(* Logix 5000 AddOnInstructionDefinition export HI6200_Faceplate_AOI; software revision 30.00; part 2 of 2 *)
(* tags used below, declared in another part *)
   Input_hi6200 : _0102:Hardy6200Series_F6857DC7:I:0;
   Output_hi6200 : _0102:Hardy6200Series_52E4DDE0:O:0;
   pm_4101 : REAL;   // Ref Weight
   pm_4182 : REAL;   // Span Weight
   pm_2082 : DINT;   // Averages
   pm_6302 : REAL;   // Auto Zero tolerance
   pm_2886 : REAL;   // Zero Tolerance
   pm_2887 : REAL;   // Motion tolerance
   pm_6183 : REAL;   // Tare Weight
   rd_filter_settings : BOOL;   // Read filter settings
   input_cmd_status : INT;   // Filtered Cmd Status
   rd_zero_tare_settings : BOOL;   // read zero and tare settings
   rd_setup1_settings : BOOL;   // read setup 1 settings
   rd_tradcal_settings : BOOL;   // program control bit to read hard cal ref weight
   write_tradcal_settings : BOOL;   // trigger write hard cal settings
   write_filter_settings : BOOL;   // trigger write filter settings
   write_zero_tare_settings : BOOL;   // trigger write zero and tare settings
   write_units_setting : BOOL;   // trigger write units of measure
   pm_2888 : REAL;   // Capacity
   rd_setup2_settings : BOOL;   // read setup 2 settings
   write_setup2_settings : BOOL;   // trigger write ins settup 2 settings
   write_setup1_settings : BOOL;   // trigger write ins setup 1 settings
   pm_2081w : DINT;   // write value setting for WAVERSAVER
   pm_6301w : DINT;   // write value setting for auto zero tracking enable
   pm_2881w : DINT;   // write value for setting units of measure
   pm_2882w : DINT;   // write value for setting decimal places
   pm_2883w : DINT;   // write value for setting grad size
   pm_4081w : DINT;   // write value for setting sensitivity value
   cmd_no : INT;   // cmd num holding register
   wr_hard_cal_ref_wt : BOOL;   // program control bit writing hard cal ref weight
   check_status_wr_traditional_ref : BOOL;   // operational code control bit write hard cal ref
   wr_span_wt : BOOL;   // program control bit writing span weight
   check_status_wr_span_wt : BOOL;   // operational code control bit write span weight
   ons_13 : BOOL;
   wr_waversaver : BOOL;   // program control bit writing WAVERSAVER
   check_status_wr_waversaver : BOOL;   // operational code control bit write WAVERSAVER
   wr_avgerages : BOOL;   // program control bit writing averages
   check_status_wr_averages : BOOL;   // operational code control bit write Averages
   wr_auto_zero_enable : BOOL;   // program control bit writing zuto zero enable
   check_status_wr_auto_zero_enable : BOOL;   // operational code control bit writing Auto Zero enable
   ons_14 : BOOL;
   wr_auto_zero_tolerance : BOOL;   // program control bit writing auto zero tolerance
   check_status_wr_auto_zero_tolerance : BOOL;   // operational code control bit writing Auto Zero tolerance
   wr_zero_tolerance : BOOL;   // program control bit writing zero tolerance
   check_status_wr_zero_tolerance : BOOL;   // operational code control bit write zero tolerance
   wr_units_measure : BOOL;   // program control bit writing units of measure
   ons_15 : BOOL;
   check_status_wr_units_measure : BOOL;   // operational code control bit write units of measure
   wr_motion_tolerance : BOOL;   // program control bit writing motion tolerance
   check_status_wr_motion_tolerance : BOOL;   // operational code control bit write motion tolerance
   wr_tare_weight : BOOL;   // program control bit writing tare weight
   check_status_wr_tare_weight : BOOL;   // operational code control bit write tare weight
   wr_sensitivity : BOOL;   // program control bit writing sensitivity
   check_status_wr_sensitivity : BOOL;   // operational code control bit write sensitivity
   wr_scale_capacity : BOOL;   // program control bit writing scale capacity
   check_status_wr_scale_capacity : BOOL;   // operational code control bit write scale capacity
   ons_17 : BOOL;
   wr_decimal_point : BOOL;   // program control bit writing decimal point
   check_status_wr_decimal_point : BOOL;   // operational code control bit writing decimal points
   wr_grad_size : BOOL;   // program control bit writing grad size
   check_status_wr_grads_size : BOOL;   // operational code control bit write grad size
   ons_18 : BOOL;
(* HI6200_Faceplate_AOI, continued *)

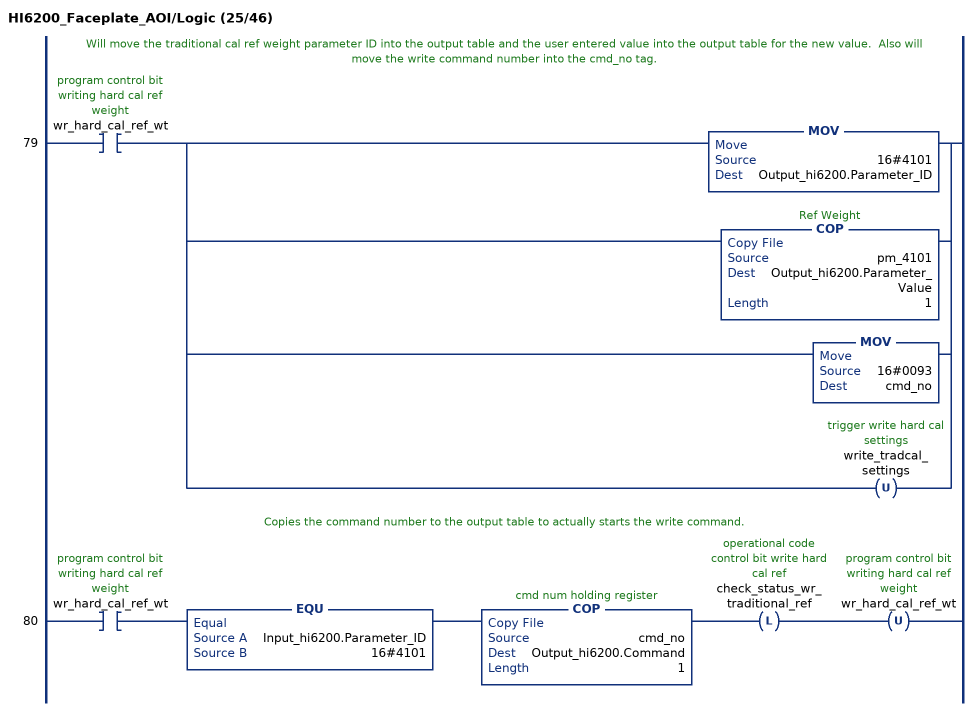
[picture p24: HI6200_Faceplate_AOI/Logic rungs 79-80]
   // Will move the traditional cal ref weight parameter ID into the output table and the user entered value into the output table for the new value.  Also will move the write command number into the cmd_no tag.
   79: XIC(wr_hard_cal_ref_wt)[MOV(16#4101,Output_hi6200.Parameter_ID) ,COP(pm_4101,Output_hi6200.Parameter_Value,1) ,MOV(16#0093,cmd_no) ,OTU(write_tradcal_settings) ];
   // Copies the command number to the output table to actually starts the write command.
   80: XIC(wr_hard_cal_ref_wt)EQU(Input_hi6200.Parameter_ID,16#4101)COP(cmd_no,Output_hi6200.Command,1)OTL(check_status_wr_traditional_ref)OTU(wr_hard_cal_ref_wt);
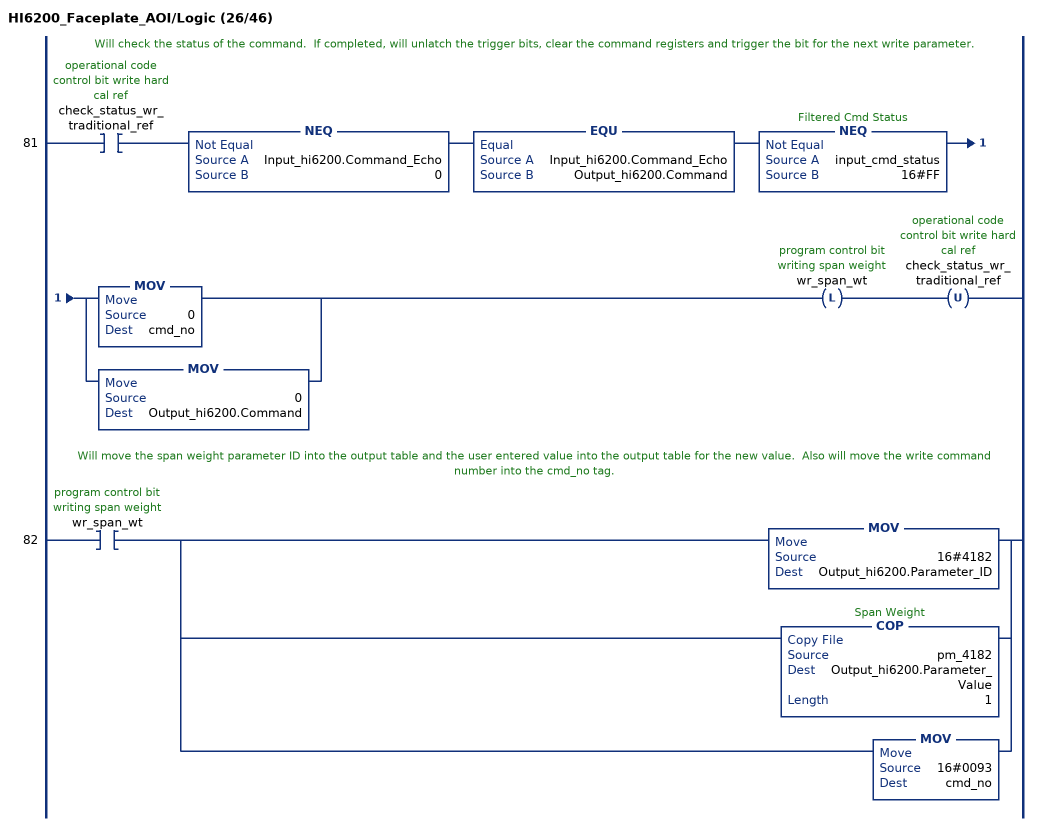
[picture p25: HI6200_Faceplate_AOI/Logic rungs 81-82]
   // Will check the status of the command.  If completed, will unlatch the trigger bits, clear the command registers and trigger the bit for the next write parameter.
   81: XIC(check_status_wr_traditional_ref)NEQ(Input_hi6200.Command_Echo,0)EQU(Input_hi6200.Command_Echo,Output_hi6200.Command)NEQ(input_cmd_status,16#FF)[MOV(0,cmd_no) ,MOV(0,Output_hi6200.Command) ]OTL(wr_span_wt)OTU(check_status_wr_traditional_ref);
   // Will move the span weight parameter ID into the output table and the user entered value into the output table for the new value.  Also will move the write command number into the cmd_no tag.
   82: XIC(wr_span_wt)[MOV(16#4182,Output_hi6200.Parameter_ID) ,COP(pm_4182,Output_hi6200.Parameter_Value,1) ,MOV(16#0093,cmd_no) ];
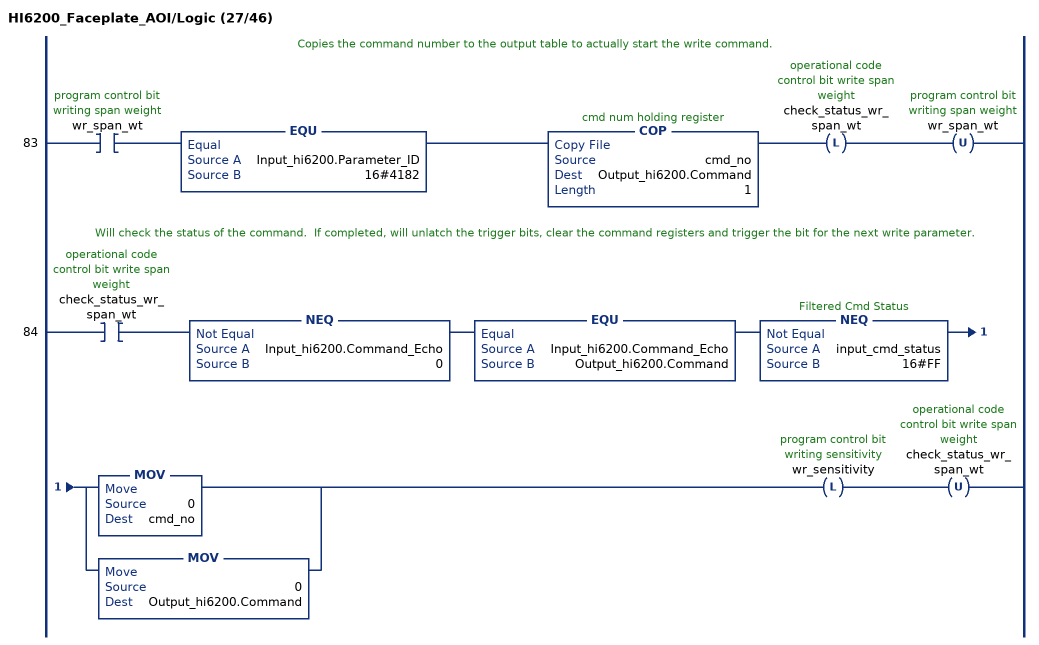
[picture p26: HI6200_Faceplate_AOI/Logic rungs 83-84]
   // Copies the command number to the output table to actually start the write command.
   83: XIC(wr_span_wt)EQU(Input_hi6200.Parameter_ID,16#4182)COP(cmd_no,Output_hi6200.Command,1)OTL(check_status_wr_span_wt)OTU(wr_span_wt);
   // Will check the status of the command.  If completed, will unlatch the trigger bits, clear the command registers and trigger the bit for the next write parameter.
   84: XIC(check_status_wr_span_wt)NEQ(Input_hi6200.Command_Echo,0)EQU(Input_hi6200.Command_Echo,Output_hi6200.Command)NEQ(input_cmd_status,16#FF)[MOV(0,cmd_no) ,MOV(0,Output_hi6200.Command) ]OTL(wr_sensitivity)OTU(check_status_wr_span_wt);
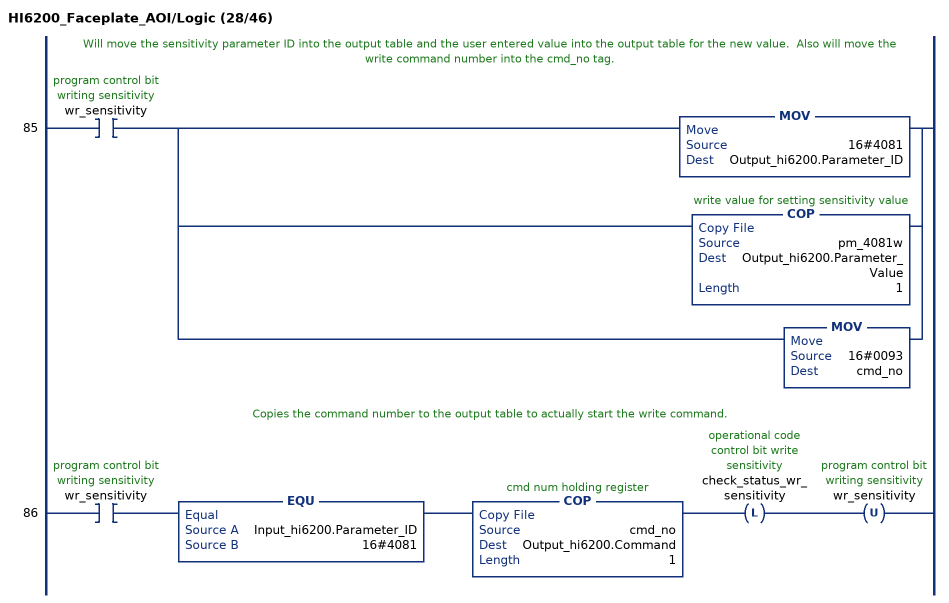
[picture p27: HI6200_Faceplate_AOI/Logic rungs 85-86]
   // Will move the sensitivity parameter ID into the output table and the user entered value into the output table for the new value.  Also will move the write command number into the cmd_no tag.
   85: XIC(wr_sensitivity)[MOV(16#4081,Output_hi6200.Parameter_ID) ,COP(pm_4081w,Output_hi6200.Parameter_Value,1) ,MOV(16#0093,cmd_no) ];
   // Copies the command number to the output table to actually start the write command.
   86: XIC(wr_sensitivity)EQU(Input_hi6200.Parameter_ID,16#4081)COP(cmd_no,Output_hi6200.Command,1)OTL(check_status_wr_sensitivity)OTU(wr_sensitivity);
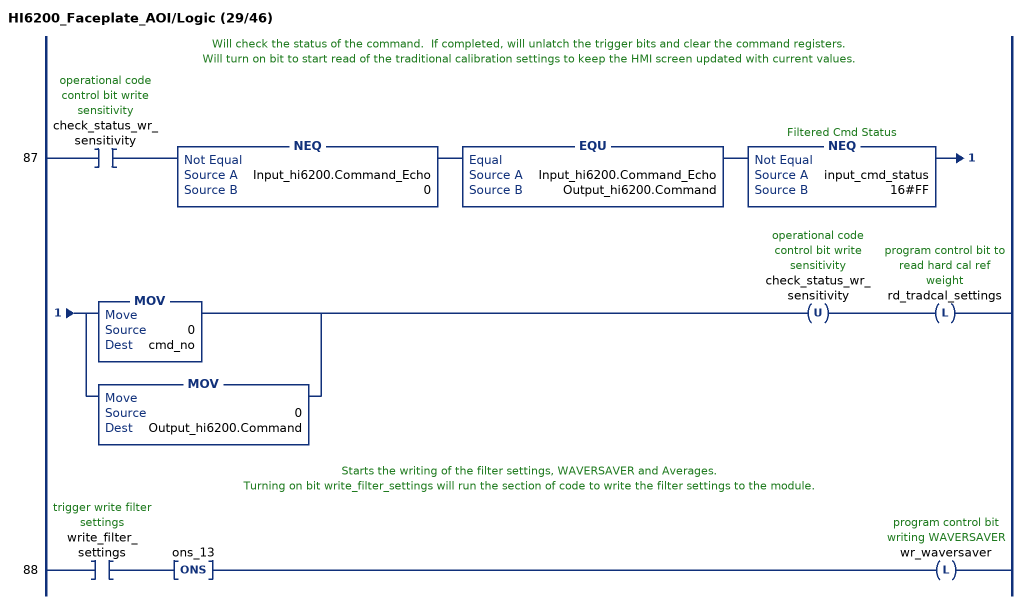
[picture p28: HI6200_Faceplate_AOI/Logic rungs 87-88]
   // Will check the status of the command.  If completed, will unlatch the trigger bits and clear the command registers.
   // Will turn on bit to start read of the traditional calibration settings to keep the HMI screen updated with current values.
   87: XIC(check_status_wr_sensitivity)NEQ(Input_hi6200.Command_Echo,0)EQU(Input_hi6200.Command_Echo,Output_hi6200.Command)NEQ(input_cmd_status,16#FF)[MOV(0,cmd_no) ,MOV(0,Output_hi6200.Command) ]OTU(check_status_wr_sensitivity)OTL(rd_tradcal_settings);
   // Starts the writing of the filter settings, WAVERSAVER and Averages.
   // Turning on bit write_filter_settings will run the section of code to write the filter settings to the module.
   88: XIC(write_filter_settings)ONS(ons_13)OTL(wr_waversaver);
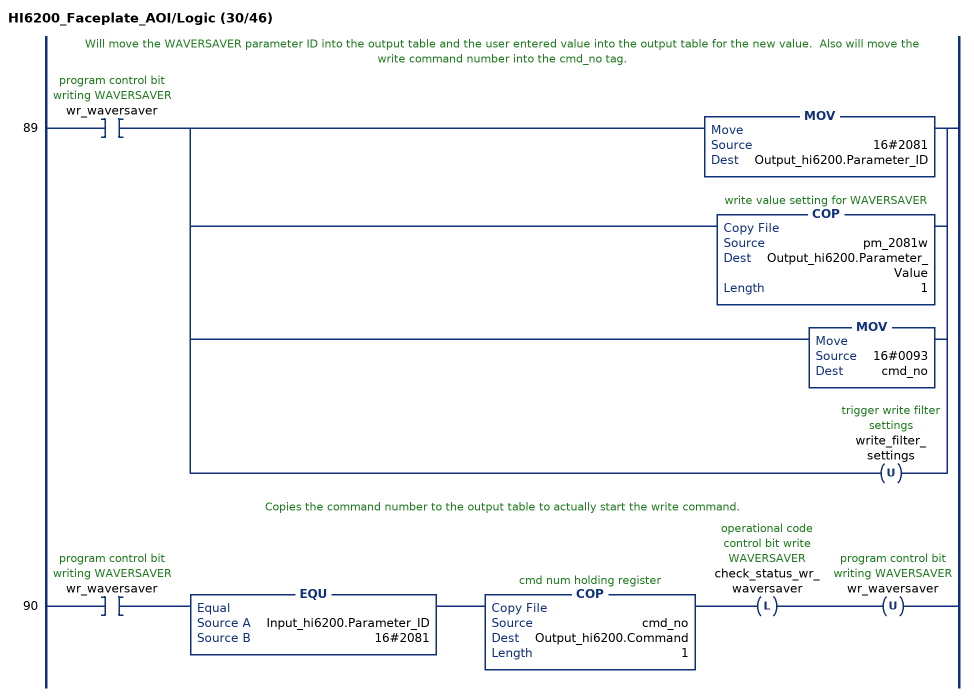
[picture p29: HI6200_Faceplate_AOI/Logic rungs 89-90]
   // Will move the WAVERSAVER parameter ID into the output table and the user entered value into the output table for the new value.  Also will move the write command number into the cmd_no tag.
   89: XIC(wr_waversaver)[MOV(16#2081,Output_hi6200.Parameter_ID) ,COP(pm_2081w,Output_hi6200.Parameter_Value,1) ,MOV(16#0093,cmd_no) ,OTU(write_filter_settings) ];
   // Copies the command number to the output table to actually start the write command.
   90: XIC(wr_waversaver)EQU(Input_hi6200.Parameter_ID,16#2081)COP(cmd_no,Output_hi6200.Command,1)OTL(check_status_wr_waversaver)OTU(wr_waversaver);
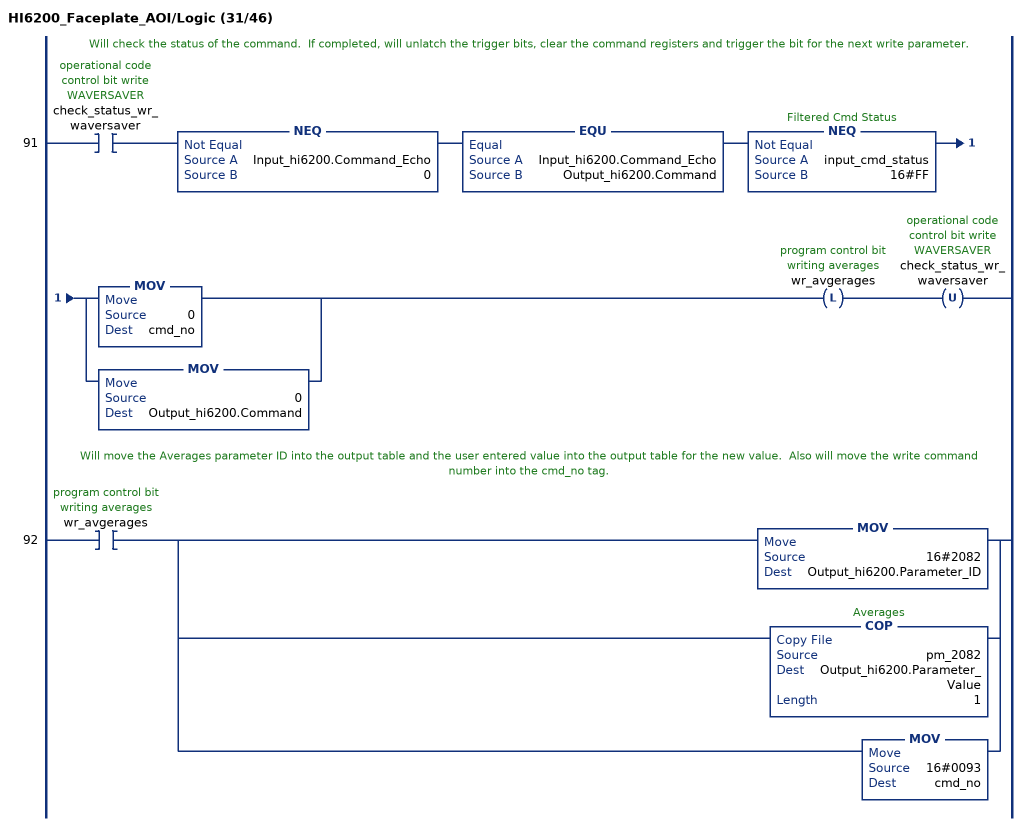
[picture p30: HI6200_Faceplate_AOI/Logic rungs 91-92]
   // Will check the status of the command.  If completed, will unlatch the trigger bits, clear the command registers and trigger the bit for the next write parameter.
   91: XIC(check_status_wr_waversaver)NEQ(Input_hi6200.Command_Echo,0)EQU(Input_hi6200.Command_Echo,Output_hi6200.Command)NEQ(input_cmd_status,16#FF)[MOV(0,cmd_no) ,MOV(0,Output_hi6200.Command) ]OTL(wr_avgerages)OTU(check_status_wr_waversaver);
   // Will move the Averages parameter ID into the output table and the user entered value into the output table for the new value.  Also will move the write command number into the cmd_no tag.
   92: XIC(wr_avgerages)[MOV(16#2082,Output_hi6200.Parameter_ID) ,COP(pm_2082,Output_hi6200.Parameter_Value,1) ,MOV(16#0093,cmd_no) ];
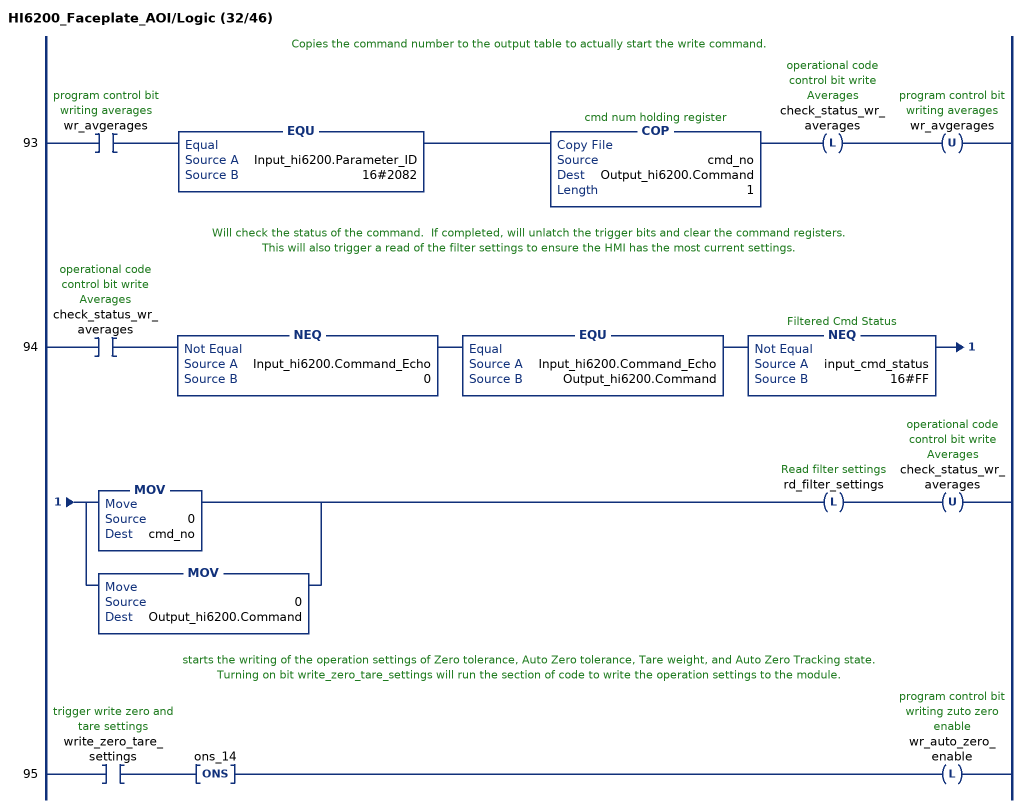
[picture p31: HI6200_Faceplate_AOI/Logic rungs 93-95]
   // Copies the command number to the output table to actually start the write command.
   93: XIC(wr_avgerages)EQU(Input_hi6200.Parameter_ID,16#2082)COP(cmd_no,Output_hi6200.Command,1)OTL(check_status_wr_averages)OTU(wr_avgerages);
   // Will check the status of the command.  If completed, will unlatch the trigger bits and clear the command registers.
   // This will also trigger a read of the filter settings to ensure the HMI has the most current settings.
   94: XIC(check_status_wr_averages)NEQ(Input_hi6200.Command_Echo,0)EQU(Input_hi6200.Command_Echo,Output_hi6200.Command)NEQ(input_cmd_status,16#FF)[MOV(0,cmd_no) ,MOV(0,Output_hi6200.Command) ]OTL(rd_filter_settings)OTU(check_status_wr_averages);
   // starts the writing of the operation settings of Zero tolerance, Auto Zero tolerance, Tare weight, and Auto Zero Tracking state.
   // Turning on bit write_zero_tare_settings will run the section of code to write the operation settings to the module.
   95: XIC(write_zero_tare_settings)ONS(ons_14)OTL(wr_auto_zero_enable);
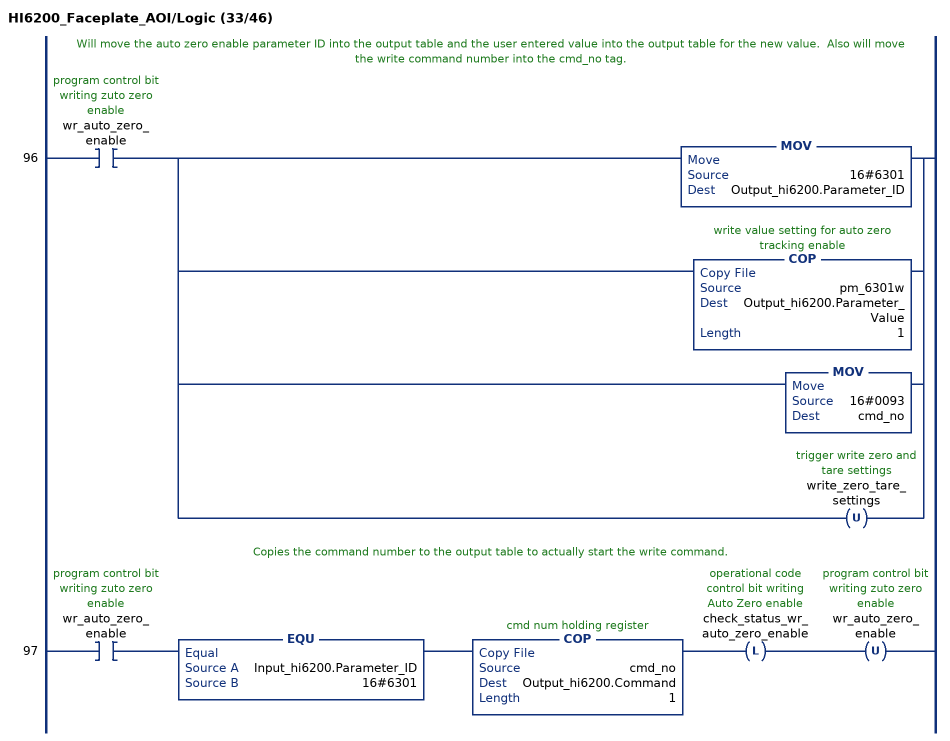
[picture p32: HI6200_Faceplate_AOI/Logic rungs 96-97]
   // Will move the auto zero enable parameter ID into the output table and the user entered value into the output table for the new value.  Also will move the write command number into the cmd_no tag.
   96: XIC(wr_auto_zero_enable)[MOV(16#6301,Output_hi6200.Parameter_ID) ,COP(pm_6301w,Output_hi6200.Parameter_Value,1) ,MOV(16#0093,cmd_no) ,OTU(write_zero_tare_settings) ];
   // Copies the command number to the output table to actually start the write command.
   97: XIC(wr_auto_zero_enable)EQU(Input_hi6200.Parameter_ID,16#6301)COP(cmd_no,Output_hi6200.Command,1)OTL(check_status_wr_auto_zero_enable)OTU(wr_auto_zero_enable);
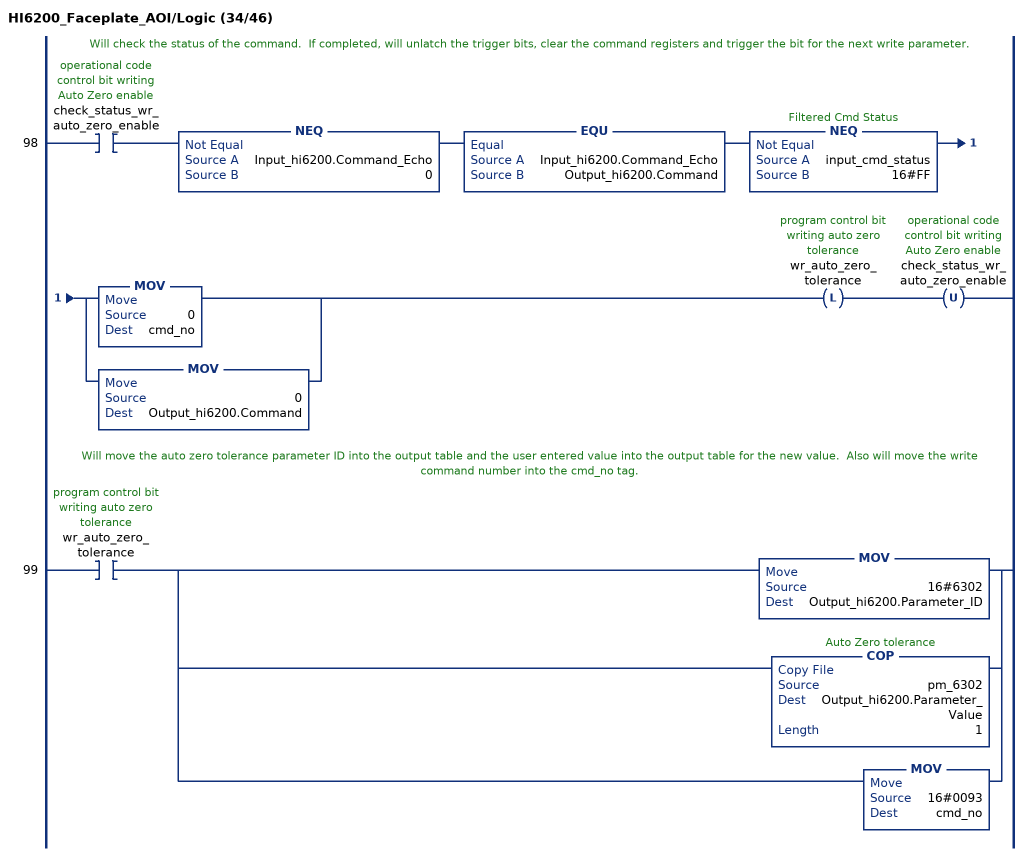
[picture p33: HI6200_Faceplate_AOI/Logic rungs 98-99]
   // Will check the status of the command.  If completed, will unlatch the trigger bits, clear the command registers and trigger the bit for the next write parameter.
   98: XIC(check_status_wr_auto_zero_enable)NEQ(Input_hi6200.Command_Echo,0)EQU(Input_hi6200.Command_Echo,Output_hi6200.Command)NEQ(input_cmd_status,16#FF)[MOV(0,cmd_no) ,MOV(0,Output_hi6200.Command) ]OTL(wr_auto_zero_tolerance)OTU(check_status_wr_auto_zero_enable);
   // Will move the auto zero tolerance parameter ID into the output table and the user entered value into the output table for the new value.  Also will move the write command number into the cmd_no tag.
   99: XIC(wr_auto_zero_tolerance)[MOV(16#6302,Output_hi6200.Parameter_ID) ,COP(pm_6302,Output_hi6200.Parameter_Value,1) ,MOV(16#0093,cmd_no) ];
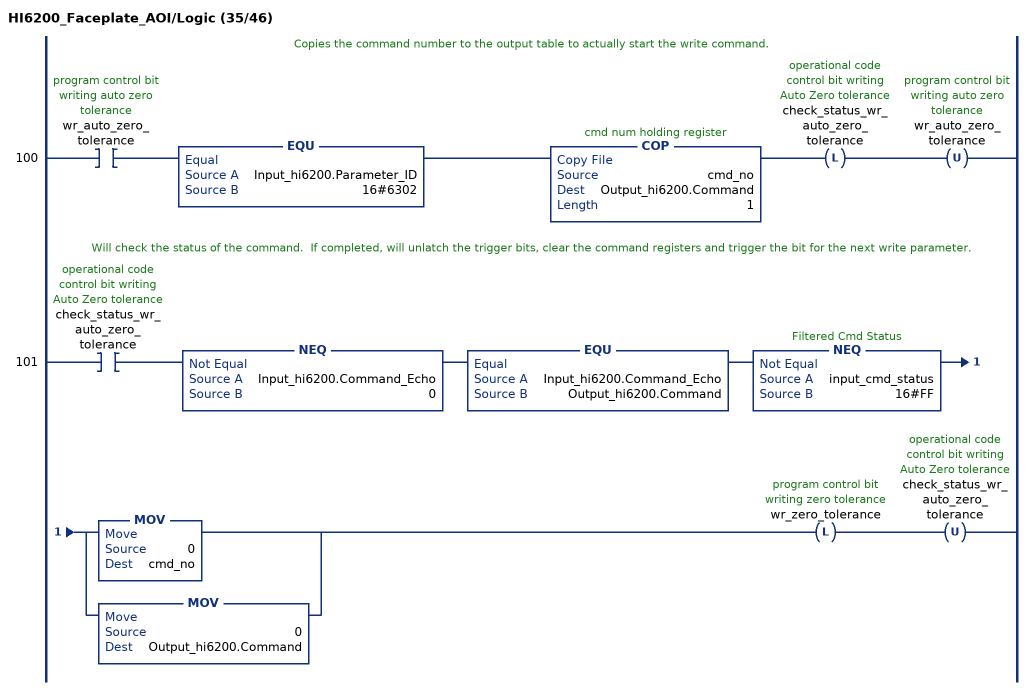
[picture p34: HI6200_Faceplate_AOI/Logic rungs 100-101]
   // Copies the command number to the output table to actually start the write command.
   100: XIC(wr_auto_zero_tolerance)EQU(Input_hi6200.Parameter_ID,16#6302)COP(cmd_no,Output_hi6200.Command,1)OTL(check_status_wr_auto_zero_tolerance)OTU(wr_auto_zero_tolerance);
   // Will check the status of the command.  If completed, will unlatch the trigger bits, clear the command registers and trigger the bit for the next write parameter.
   101: XIC(check_status_wr_auto_zero_tolerance)NEQ(Input_hi6200.Command_Echo,0)EQU(Input_hi6200.Command_Echo,Output_hi6200.Command)NEQ(input_cmd_status,16#FF)[MOV(0,cmd_no) ,MOV(0,Output_hi6200.Command) ]OTL(wr_zero_tolerance)OTU(check_status_wr_auto_zero_tolerance);
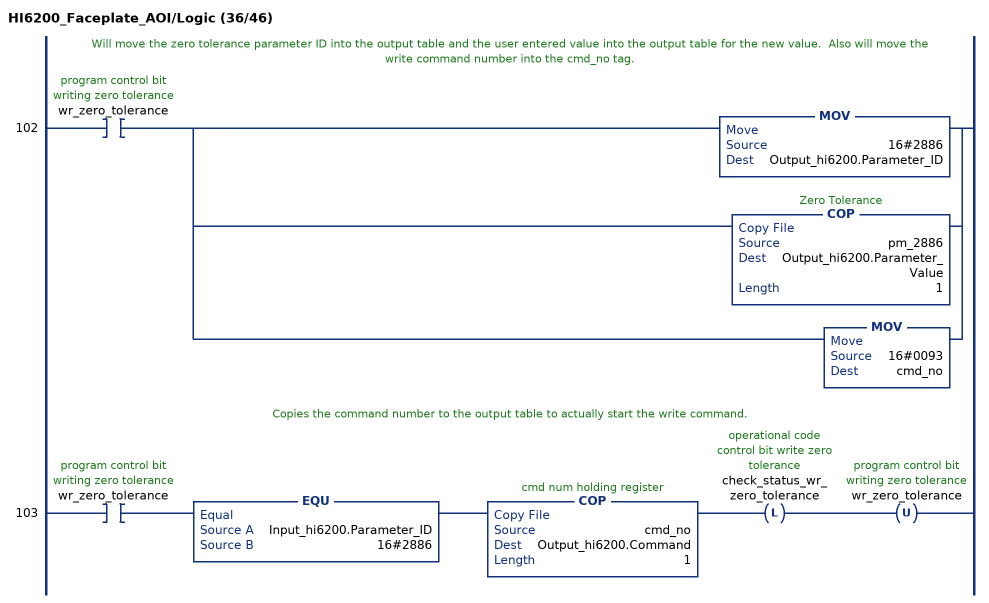
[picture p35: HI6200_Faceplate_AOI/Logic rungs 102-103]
   // Will move the zero tolerance parameter ID into the output table and the user entered value into the output table for the new value.  Also will move the write command number into the cmd_no tag.
   102: XIC(wr_zero_tolerance)[MOV(16#2886,Output_hi6200.Parameter_ID) ,COP(pm_2886,Output_hi6200.Parameter_Value,1) ,MOV(16#0093,cmd_no) ];
   // Copies the command number to the output table to actually start the write command.
   103: XIC(wr_zero_tolerance)EQU(Input_hi6200.Parameter_ID,16#2886)COP(cmd_no,Output_hi6200.Command,1)OTL(check_status_wr_zero_tolerance)OTU(wr_zero_tolerance);
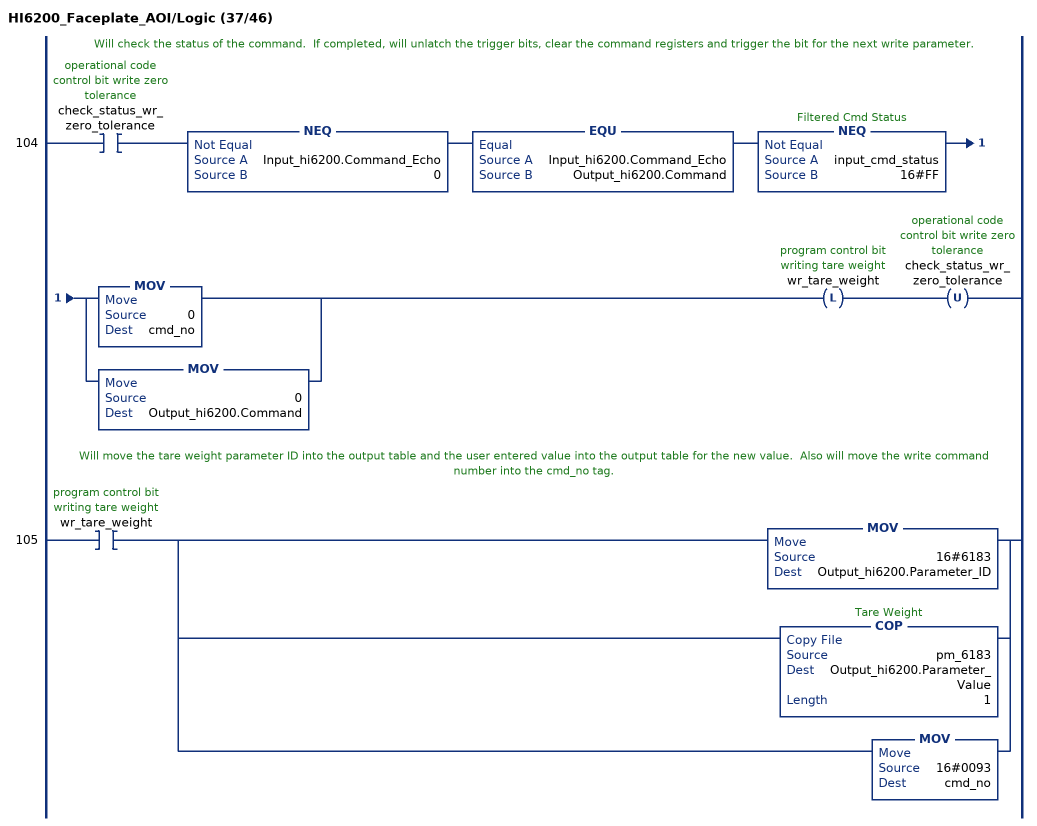
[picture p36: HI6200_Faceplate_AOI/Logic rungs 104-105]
   // Will check the status of the command.  If completed, will unlatch the trigger bits, clear the command registers and trigger the bit for the next write parameter.
   104: XIC(check_status_wr_zero_tolerance)NEQ(Input_hi6200.Command_Echo,0)EQU(Input_hi6200.Command_Echo,Output_hi6200.Command)NEQ(input_cmd_status,16#FF)[MOV(0,cmd_no) ,MOV(0,Output_hi6200.Command) ]OTL(wr_tare_weight)OTU(check_status_wr_zero_tolerance);
   // Will move the tare weight parameter ID into the output table and the user entered value into the output table for the new value.  Also will move the write command number into the cmd_no tag.
   105: XIC(wr_tare_weight)[MOV(16#6183,Output_hi6200.Parameter_ID) ,COP(pm_6183,Output_hi6200.Parameter_Value,1) ,MOV(16#0093,cmd_no) ];
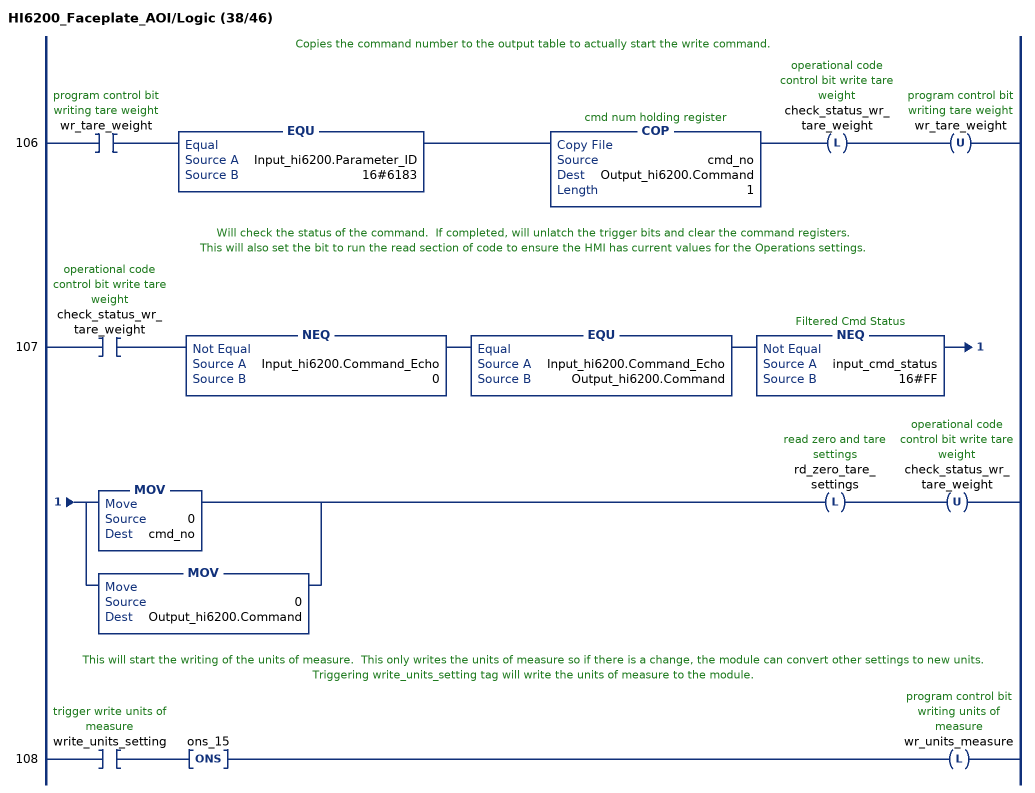
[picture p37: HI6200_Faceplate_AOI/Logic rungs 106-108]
   // Copies the command number to the output table to actually start the write command.
   106: XIC(wr_tare_weight)EQU(Input_hi6200.Parameter_ID,16#6183)COP(cmd_no,Output_hi6200.Command,1)OTL(check_status_wr_tare_weight)OTU(wr_tare_weight);
   // Will check the status of the command.  If completed, will unlatch the trigger bits and clear the command registers.
   // This will also set the bit to run the read section of code to ensure the HMI has current values for the Operations settings.
   107: XIC(check_status_wr_tare_weight)NEQ(Input_hi6200.Command_Echo,0)EQU(Input_hi6200.Command_Echo,Output_hi6200.Command)NEQ(input_cmd_status,16#FF)[MOV(0,cmd_no) ,MOV(0,Output_hi6200.Command) ]OTL(rd_zero_tare_settings)OTU(check_status_wr_tare_weight);
   // This will start the writing of the units of measure.  This only writes the units of measure so if there is a change, the module can convert other settings to new units.
   // Triggering write_units_setting tag will write the units of measure to the module.
   108: XIC(write_units_setting)ONS(ons_15)OTL(wr_units_measure);
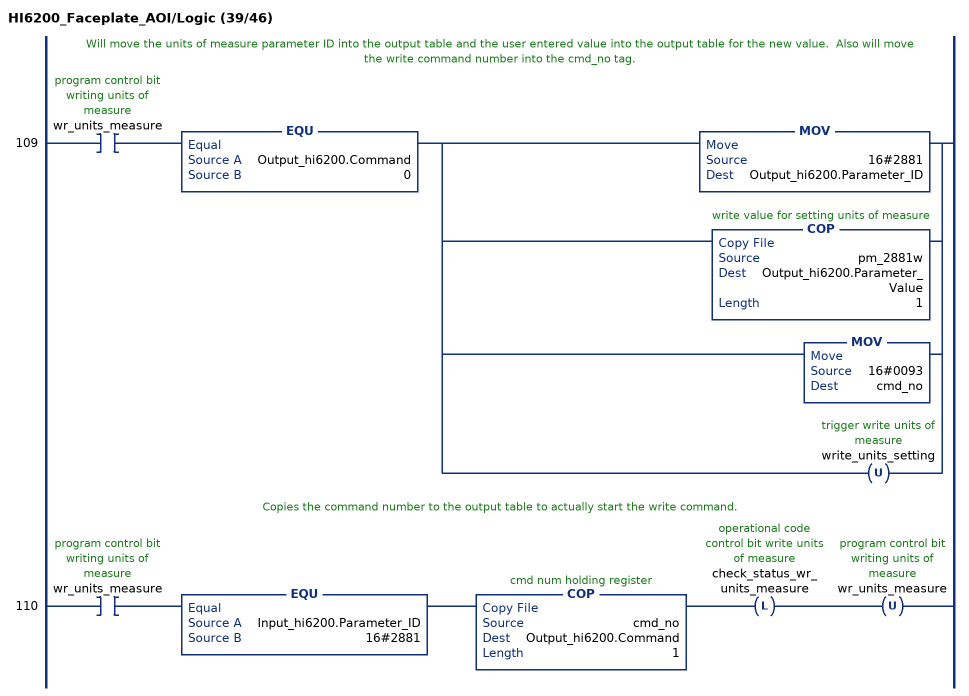
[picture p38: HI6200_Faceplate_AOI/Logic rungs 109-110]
   // Will move the units of measure parameter ID into the output table and the user entered value into the output table for the new value.  Also will move the write command number into the cmd_no tag.
   109: XIC(wr_units_measure)EQU(Output_hi6200.Command,0)[MOV(16#2881,Output_hi6200.Parameter_ID) ,COP(pm_2881w,Output_hi6200.Parameter_Value,1) ,MOV(16#0093,cmd_no) ,OTU(write_units_setting) ];
   // Copies the command number to the output table to actually start the write command.
   110: XIC(wr_units_measure)EQU(Input_hi6200.Parameter_ID,16#2881)COP(cmd_no,Output_hi6200.Command,1)OTL(check_status_wr_units_measure)OTU(wr_units_measure);
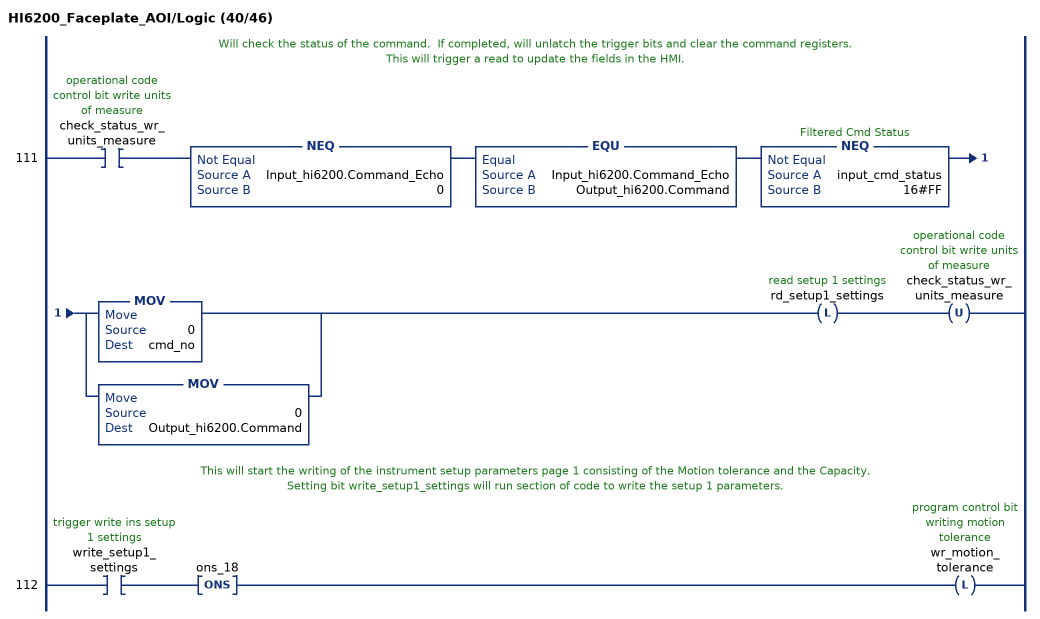
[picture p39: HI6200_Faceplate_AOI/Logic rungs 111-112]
   // Will check the status of the command.  If completed, will unlatch the trigger bits and clear the command registers.
   // This will trigger a read to update the fields in the HMI.
   111: XIC(check_status_wr_units_measure)NEQ(Input_hi6200.Command_Echo,0)EQU(Input_hi6200.Command_Echo,Output_hi6200.Command)NEQ(input_cmd_status,16#FF)[MOV(0,cmd_no) ,MOV(0,Output_hi6200.Command) ]OTL(rd_setup1_settings)OTU(check_status_wr_units_measure);
   // This will start the writing of the instrument setup parameters page 1 consisting of the Motion tolerance and the Capacity.
   // Setting bit write_setup1_settings will run section of code to write the setup 1 parameters.
   112: XIC(write_setup1_settings)ONS(ons_18)OTL(wr_motion_tolerance);
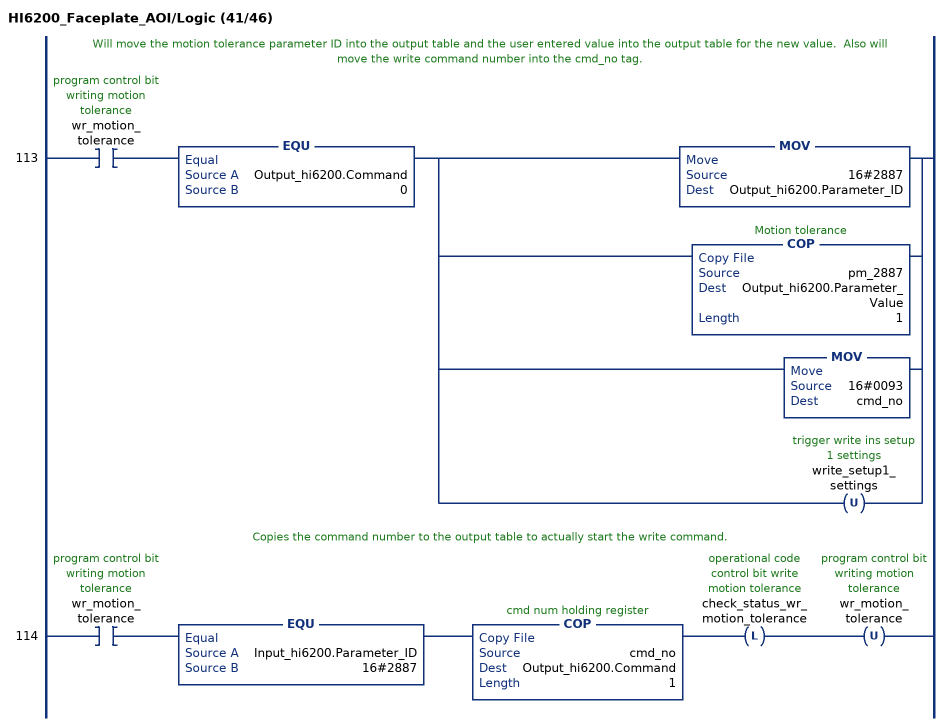
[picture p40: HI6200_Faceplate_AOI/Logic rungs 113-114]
   // Will move the motion tolerance parameter ID into the output table and the user entered value into the output table for the new value.  Also will move the write command number into the cmd_no tag.
   113: XIC(wr_motion_tolerance)EQU(Output_hi6200.Command,0)[MOV(16#2887,Output_hi6200.Parameter_ID) ,COP(pm_2887,Output_hi6200.Parameter_Value,1) ,MOV(16#0093,cmd_no) ,OTU(write_setup1_settings) ];
   // Copies the command number to the output table to actually start the write command.
   114: XIC(wr_motion_tolerance)EQU(Input_hi6200.Parameter_ID,16#2887)COP(cmd_no,Output_hi6200.Command,1)OTL(check_status_wr_motion_tolerance)OTU(wr_motion_tolerance);
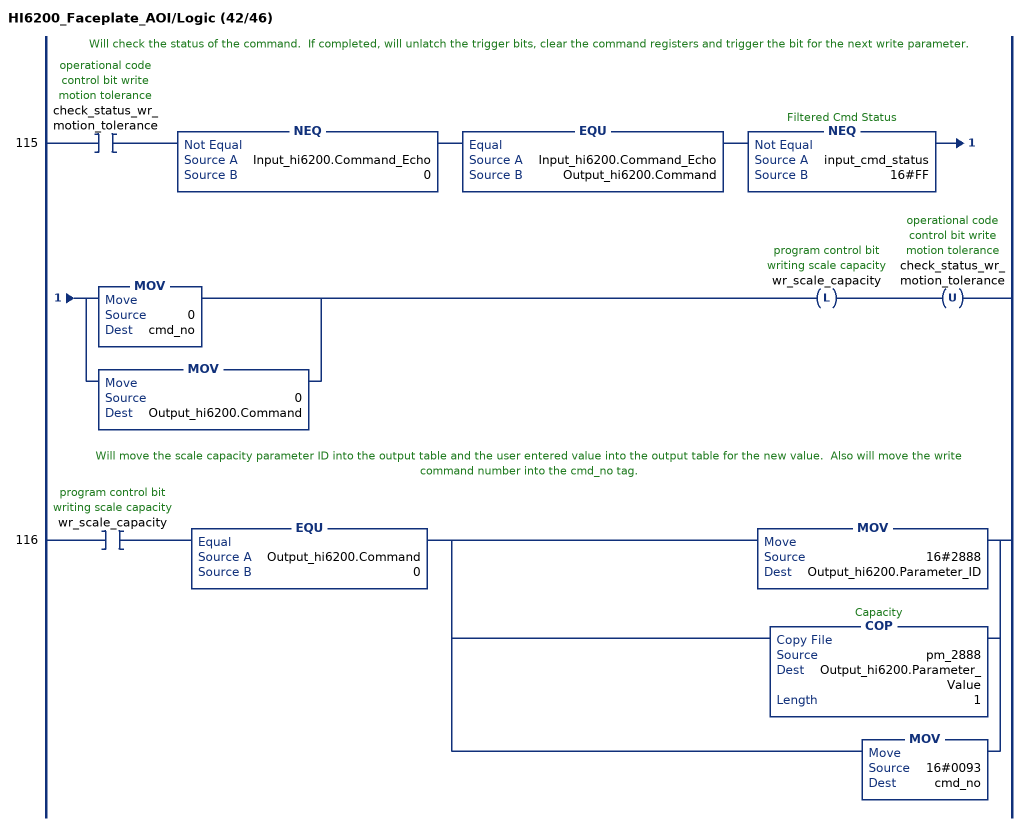
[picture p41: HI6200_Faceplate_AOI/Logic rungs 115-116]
   // Will check the status of the command.  If completed, will unlatch the trigger bits, clear the command registers and trigger the bit for the next write parameter.
   115: XIC(check_status_wr_motion_tolerance)NEQ(Input_hi6200.Command_Echo,0)EQU(Input_hi6200.Command_Echo,Output_hi6200.Command)NEQ(input_cmd_status,16#FF)[MOV(0,cmd_no) ,MOV(0,Output_hi6200.Command) ]OTL(wr_scale_capacity)OTU(check_status_wr_motion_tolerance);
   // Will move the scale capacity parameter ID into the output table and the user entered value into the output table for the new value.  Also will move the write command number into the cmd_no tag.
   116: XIC(wr_scale_capacity)EQU(Output_hi6200.Command,0)[MOV(16#2888,Output_hi6200.Parameter_ID) ,COP(pm_2888,Output_hi6200.Parameter_Value,1) ,MOV(16#0093,cmd_no) ];
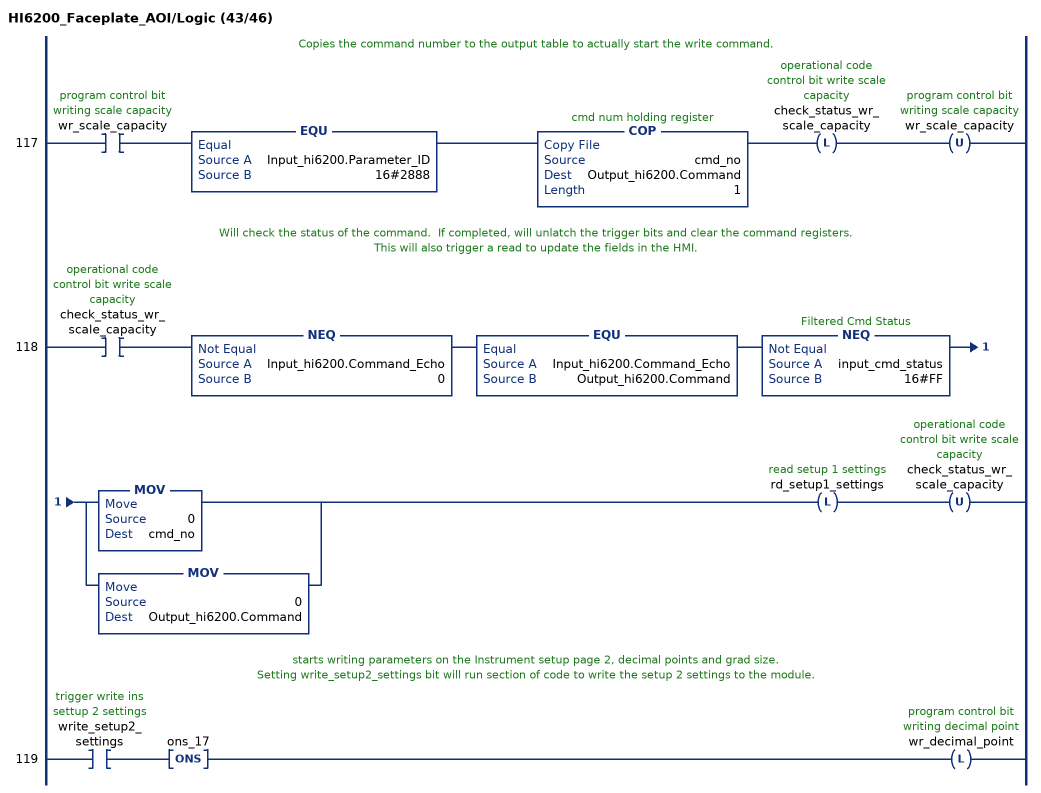
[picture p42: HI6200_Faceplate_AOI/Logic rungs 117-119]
   // Copies the command number to the output table to actually start the write command.
   117: XIC(wr_scale_capacity)EQU(Input_hi6200.Parameter_ID,16#2888)COP(cmd_no,Output_hi6200.Command,1)OTL(check_status_wr_scale_capacity)OTU(wr_scale_capacity);
   // Will check the status of the command.  If completed, will unlatch the trigger bits and clear the command registers.
   // This will also trigger a read to update the fields in the HMI.
   118: XIC(check_status_wr_scale_capacity)NEQ(Input_hi6200.Command_Echo,0)EQU(Input_hi6200.Command_Echo,Output_hi6200.Command)NEQ(input_cmd_status,16#FF)[MOV(0,cmd_no) ,MOV(0,Output_hi6200.Command) ]OTL(rd_setup1_settings)OTU(check_status_wr_scale_capacity);
   // starts writing parameters on the Instrument setup page 2, decimal points and grad size.
   // Setting write_setup2_settings bit will run section of code to write the setup 2 settings to the module.
   119: XIC(write_setup2_settings)ONS(ons_17)OTL(wr_decimal_point);
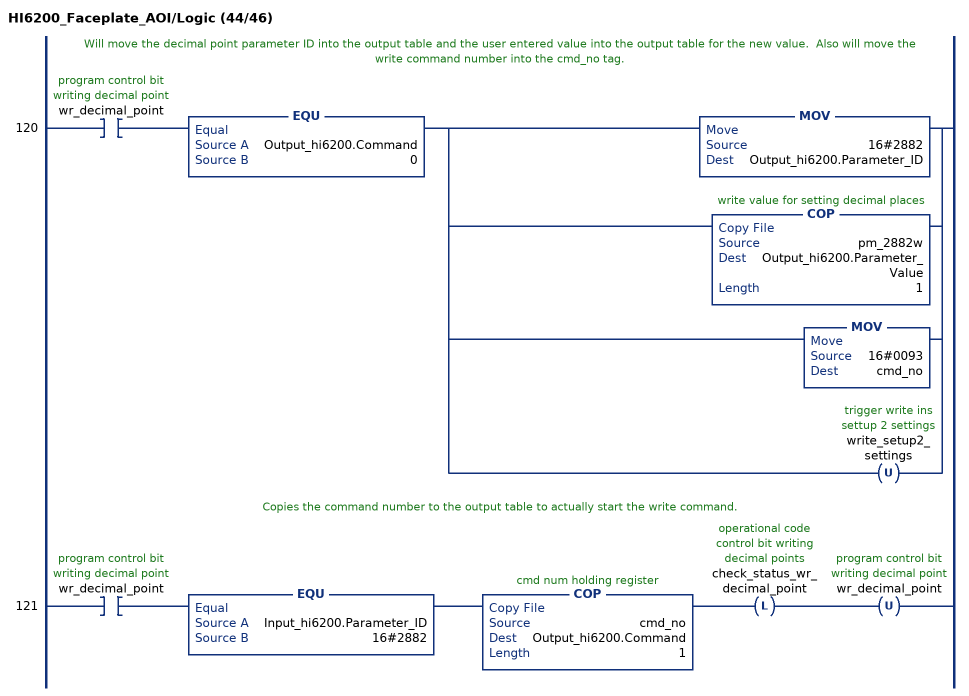
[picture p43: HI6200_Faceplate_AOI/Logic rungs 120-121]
   // Will move the decimal point parameter ID into the output table and the user entered value into the output table for the new value.  Also will move the write command number into the cmd_no tag.
   120: XIC(wr_decimal_point)EQU(Output_hi6200.Command,0)[MOV(16#2882,Output_hi6200.Parameter_ID) ,COP(pm_2882w,Output_hi6200.Parameter_Value,1) ,MOV(16#0093,cmd_no) ,OTU(write_setup2_settings) ];
   // Copies the command number to the output table to actually start the write command.
   121: XIC(wr_decimal_point)EQU(Input_hi6200.Parameter_ID,16#2882)COP(cmd_no,Output_hi6200.Command,1)OTL(check_status_wr_decimal_point)OTU(wr_decimal_point);
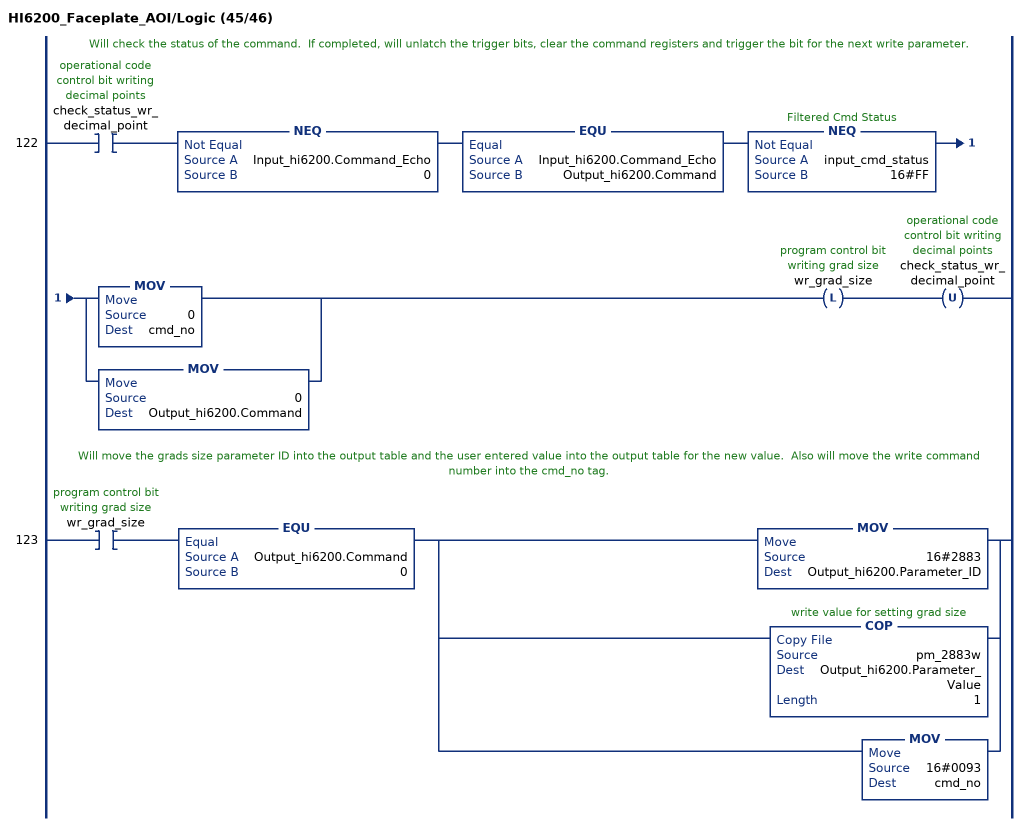
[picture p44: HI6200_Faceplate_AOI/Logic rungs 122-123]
   // Will check the status of the command.  If completed, will unlatch the trigger bits, clear the command registers and trigger the bit for the next write parameter.
   122: XIC(check_status_wr_decimal_point)NEQ(Input_hi6200.Command_Echo,0)EQU(Input_hi6200.Command_Echo,Output_hi6200.Command)NEQ(input_cmd_status,16#FF)[MOV(0,cmd_no) ,MOV(0,Output_hi6200.Command) ]OTL(wr_grad_size)OTU(check_status_wr_decimal_point);
   // Will move the grads size parameter ID into the output table and the user entered value into the output table for the new value.  Also will move the write command number into the cmd_no tag.
   123: XIC(wr_grad_size)EQU(Output_hi6200.Command,0)[MOV(16#2883,Output_hi6200.Parameter_ID) ,COP(pm_2883w,Output_hi6200.Parameter_Value,1) ,MOV(16#0093,cmd_no) ];
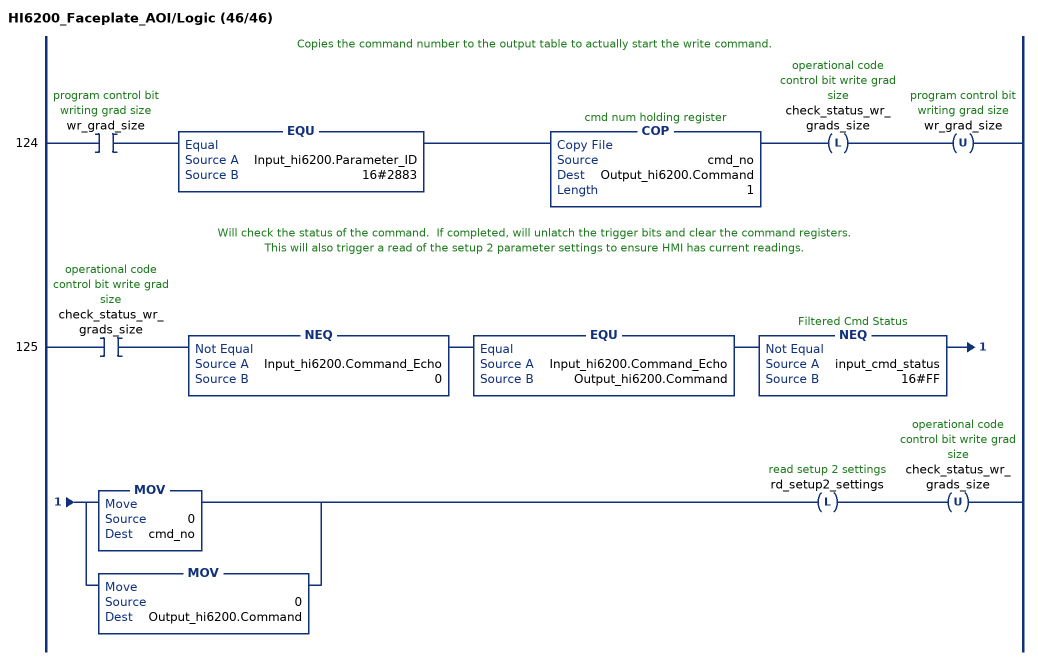
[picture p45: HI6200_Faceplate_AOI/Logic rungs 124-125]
   // Copies the command number to the output table to actually start the write command.
   124: XIC(wr_grad_size)EQU(Input_hi6200.Parameter_ID,16#2883)COP(cmd_no,Output_hi6200.Command,1)OTL(check_status_wr_grads_size)OTU(wr_grad_size);
   // Will check the status of the command.  If completed, will unlatch the trigger bits and clear the command registers.
   // This will also trigger a read of the setup 2 parameter settings to ensure HMI has current readings.
   125: XIC(check_status_wr_grads_size)NEQ(Input_hi6200.Command_Echo,0)EQU(Input_hi6200.Command_Echo,Output_hi6200.Command)NEQ(input_cmd_status,16#FF)[MOV(0,cmd_no) ,MOV(0,Output_hi6200.Command) ]OTL(rd_setup2_settings)OTU(check_status_wr_grads_size);
END_ROUTINE
END_ADD_ON_INSTRUCTION
